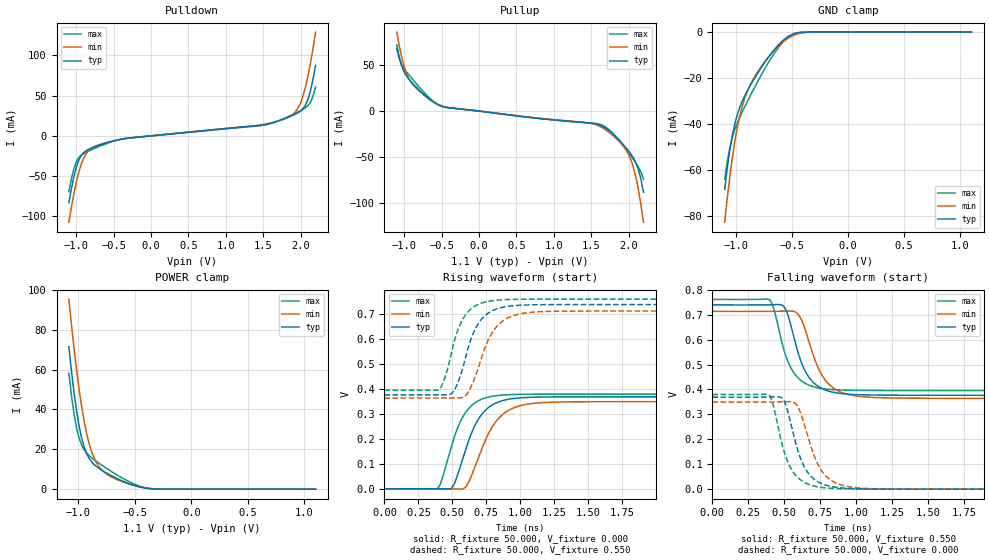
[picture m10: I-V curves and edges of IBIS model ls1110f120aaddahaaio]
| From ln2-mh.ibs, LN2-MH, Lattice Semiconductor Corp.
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|   Model ls1110f120aaddahaaio
[Model] ls1110f120aaddahaaio
| Clamp models do not include dynamic input termination. Please refer to
| the ls1110axxxaaddahaain model for input termination.
Model_type I/O
Polarity   Non-Inverting
Enable   Active-Low
Vinl =  0.200V
Vinh =  0.300V
Vmeas =  0.550V
Cref =  20.000pF
Rref =  50.000
Vref =  0.600V
C_comp   2.000pF   1.500pF   2.500pF
[Temperature Range]   25.000   0.125k   -40.000
[Voltage Range]   1.100V   1.070V   1.130V
[C Comp Corner]
C_comp   2.000pF   1.500pF   2.500pF
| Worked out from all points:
|   slope of the pulldown table from 0 to 0.165 V, typ, clamps not added: 108 ohm
|   slope of the pullup table from 0 to 0.165 V, typ, clamps not added: 95.2 ohm
|   GND clamp passes 1 mA (typ) near -0.50 V on its own axis
|   POWER clamp passes 1 mA (typ) near -0.45 V on its own axis
|   rising waveform, R_fixture 50.000, V_fixture 0.000: 20-80 % time 162ps typ, 183ps min, 150ps max; typ from 0 V to 0.369 V
|   rising waveform, R_fixture 50.000, V_fixture 0.550: 20-80 % time 140ps typ, 159ps min, 127ps max; typ from 0.377 V to 0.739 V
|   falling waveform, R_fixture 50.000, V_fixture 0.550: 20-80 % time 130ps typ, 147ps min, 121ps max; typ from 0.739 V to 0.377 V
|   falling waveform, R_fixture 50.000, V_fixture 0.000: 20-80 % time 123ps typ, 136ps min, 117ps max; typ from 0.369 V to 0 V
[Pulldown]
|Voltage   I(typ)   I(min)   I(max)
-1.1V     -83.17mA   -107.2mA   -69.44mA
-1.032V   -50.45mA   -71.54mA   -40.61mA
-930mV    -23.9mA    -33.9mA    -23.62mA
-862mV    -18.05mA   -21.29mA   -20mA
-760mV    -13.75mA   -13.42mA   -15.74mA
-352mV    -3.405mA   -3.591mA   -3.262mA
1.518V    14.06mA    14.41mA    13.46mA
1.892V    25.3mA     26.48mA    26.4mA
1.994V    30.4mA     39.74mA    31.14mA
2.062V    37.79mA    59.46mA    34.81mA
2.13V     55.42mA    89.57mA    41.52mA
2.2V      87.69mA    128.9mA    60.76mA
[Pullup]
|Voltage   I(typ)   I(min)   I(max)
-1.1V     71.68mA    85.61mA    67.47mA
-1.03V    47.83mA    56.93mA    49.31mA
-928mV    33.42mA    33.98mA    38.33mA
-792mV    22.03mA    21.13mA    25.32mA
-554mV    6.994mA    7.569mA    7.286mA
1.486V    -13.06mA   -13.14mA   -12.99mA
1.724V    -20.14mA   -22.11mA   -19.26mA
1.928V    -36.24mA   -37.97mA   -37.39mA
2.03V     -46.41mA   -52.61mA   -48.41mA
2.098V    -55.96mA   -71.57mA   -56.29mA
2.166V    -73.86mA   -101.6mA   -66.17mA
2.2V      -88.05mA   -120.5mA   -73.84mA
[GND_clamp]
|Voltage   I(typ)   I(min)   I(max)
-1.1V     -68.65mA   -82.91mA   -64.16mA
-1.054V   -51.26mA   -62.87mA   -50.37mA
-1.008V   -39.63mA   -47.13mA   -42.26mA
-962mV    -32.34mA   -35.82mA   -36.73mA
-916mV    -27.28mA   -28.13mA   -32.02mA
-847mV    -21.22mA   -20.63mA   -25.4mA
-778mV    -15.81mA   -15.27mA   -19.09mA
-663mV    -7.926mA   -8.201mA   -9.607mA
-571mV    -3.246mA   -3.982mA   -3.828mA
-502mV    -1.097mA   -1.819mA   -1.164mA
-410mV    -96.97uA   -374.9uA   -57.53uA
1.1V      0A         0A         0A
[POWER_clamp]
|Voltage   I(typ)   I(min)   I(max)
-1.085V   71.41mA    95.35mA    58.18mA
-1.062V   59.23mA    82.55mA    46.99mA
-1.039V   48.36mA    70.56mA    37.71mA
-1.016V   38.97mA    59.53mA    30.53mA
-970mV    25.17mA    40.76mA    21.88mA
-924mV    17.37mA    26.93mA    17.87mA
-901mV    15.03mA    21.86mA    16.59mA
-855mV    12.01mA    14.79mA    14.5mA
-763mV    8.448mA    8.108mA    10.89mA
-533mV    2.369mA    2.267mA    3.272mA
-349mV    143.9uA    291.4uA    171.3uA
1.1V      0A         0A         0A
[Ramp]
| variable   typ   min   max
dV/dt_r   0.221/0.163n   0.210/0.183n   0.228/0.150n
dV/dt_f   0.207/0.143n   0.203/0.168n   0.205/0.131n
R_load = 50.000
[Rising Waveform]
R_fixture = 50.000
V_fixture = 0.000
V_fixture_min = 0.000
V_fixture_max = 0.000
|  time   V(typ)   V(min)   V(max)
0s        2.818uV    12.02uV    614.4nV
393ps     251.4uV    144uV      3.005mV
499ps     6.024mV    -128.1uV   179.4mV
586ps     136.4mV    1.762mV    297.1mV
711ps     294.7mV    151.9mV    358.3mV
789ps     334.8mV    244.2mV    370.6mV
881ps     355.4mV    302.8mV    376.4mV
1.04ns    366.2mV    338.3mV    379.2mV
1.36ns    368.9mV    348.8mV    379.9mV
10ns      369mV      349.6mV    379.9mV
[Rising Waveform]
R_fixture = 50.000
V_fixture = 0.550
V_fixture_min = 0.534
V_fixture_max = 0.568
|  time   V(typ)   V(min)   V(max)
0s        376.7mV    364.2mV    395.6mV
404ps     376.8mV    364.3mV    399mV
457ps     377mV      364.4mV    467.1mV
511ps     393.2mV    364.2mV    584.8mV
590ps     511.5mV    370.9mV    692mV
697ps     667.5mV    495.3mV    741.4mV
768ps     706.3mV    601.5mV    752.5mV
859ps     726.9mV    668.2mV    758.1mV
1.313ns   739mV      712.7mV    761.1mV
10ns      739.2mV    713.4mV    761.2mV
[Falling Waveform]
R_fixture = 50.000
V_fixture = 0.550
V_fixture_min = 0.534
V_fixture_max = 0.568
|  time   V(typ)   V(min)   V(max)
0s        739.2mV    713.4mV    761.2mV
399ps     739.4mV    713.4mV    758.5mV
430ps     740mV      713.5mV    717.7mV
501ps     728.9mV    714.3mV    551.6mV
582ps     576.3mV    709mV      455.3mV
678ps     443.8mV    579mV      415.7mV
753ps     406.4mV    466.2mV    404.6mV
838ps     389.1mV    407.2mV    399.4mV
1.353ns   376.9mV    365.1mV    395.7mV
10ns      376.7mV    364.2mV    395.6mV
[Falling Waveform]
R_fixture = 50.000
V_fixture = 0.000
V_fixture_min = 0.000
V_fixture_max = 0.000
|  time   V(typ)   V(min)   V(max)
0s        369mV      349.6mV    379.9mV
395ps     369.6mV    349.6mV    376.7mV
495ps     357.8mV    351mV      158.3mV
573ps     199.2mV    345.1mV    59.91mV
613ps     123.4mV    306.6mV    37.08mV
668ps     63.2mV     203mV      19.47mV
743ps     26.55mV    89.57mV    8.319mV
823ps     10.96mV    36.23mV    3.499mV
1.268ns   237.5uV    646.8uV    100.5uV
10ns      2.818uV    12.02uV    614.4nV
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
